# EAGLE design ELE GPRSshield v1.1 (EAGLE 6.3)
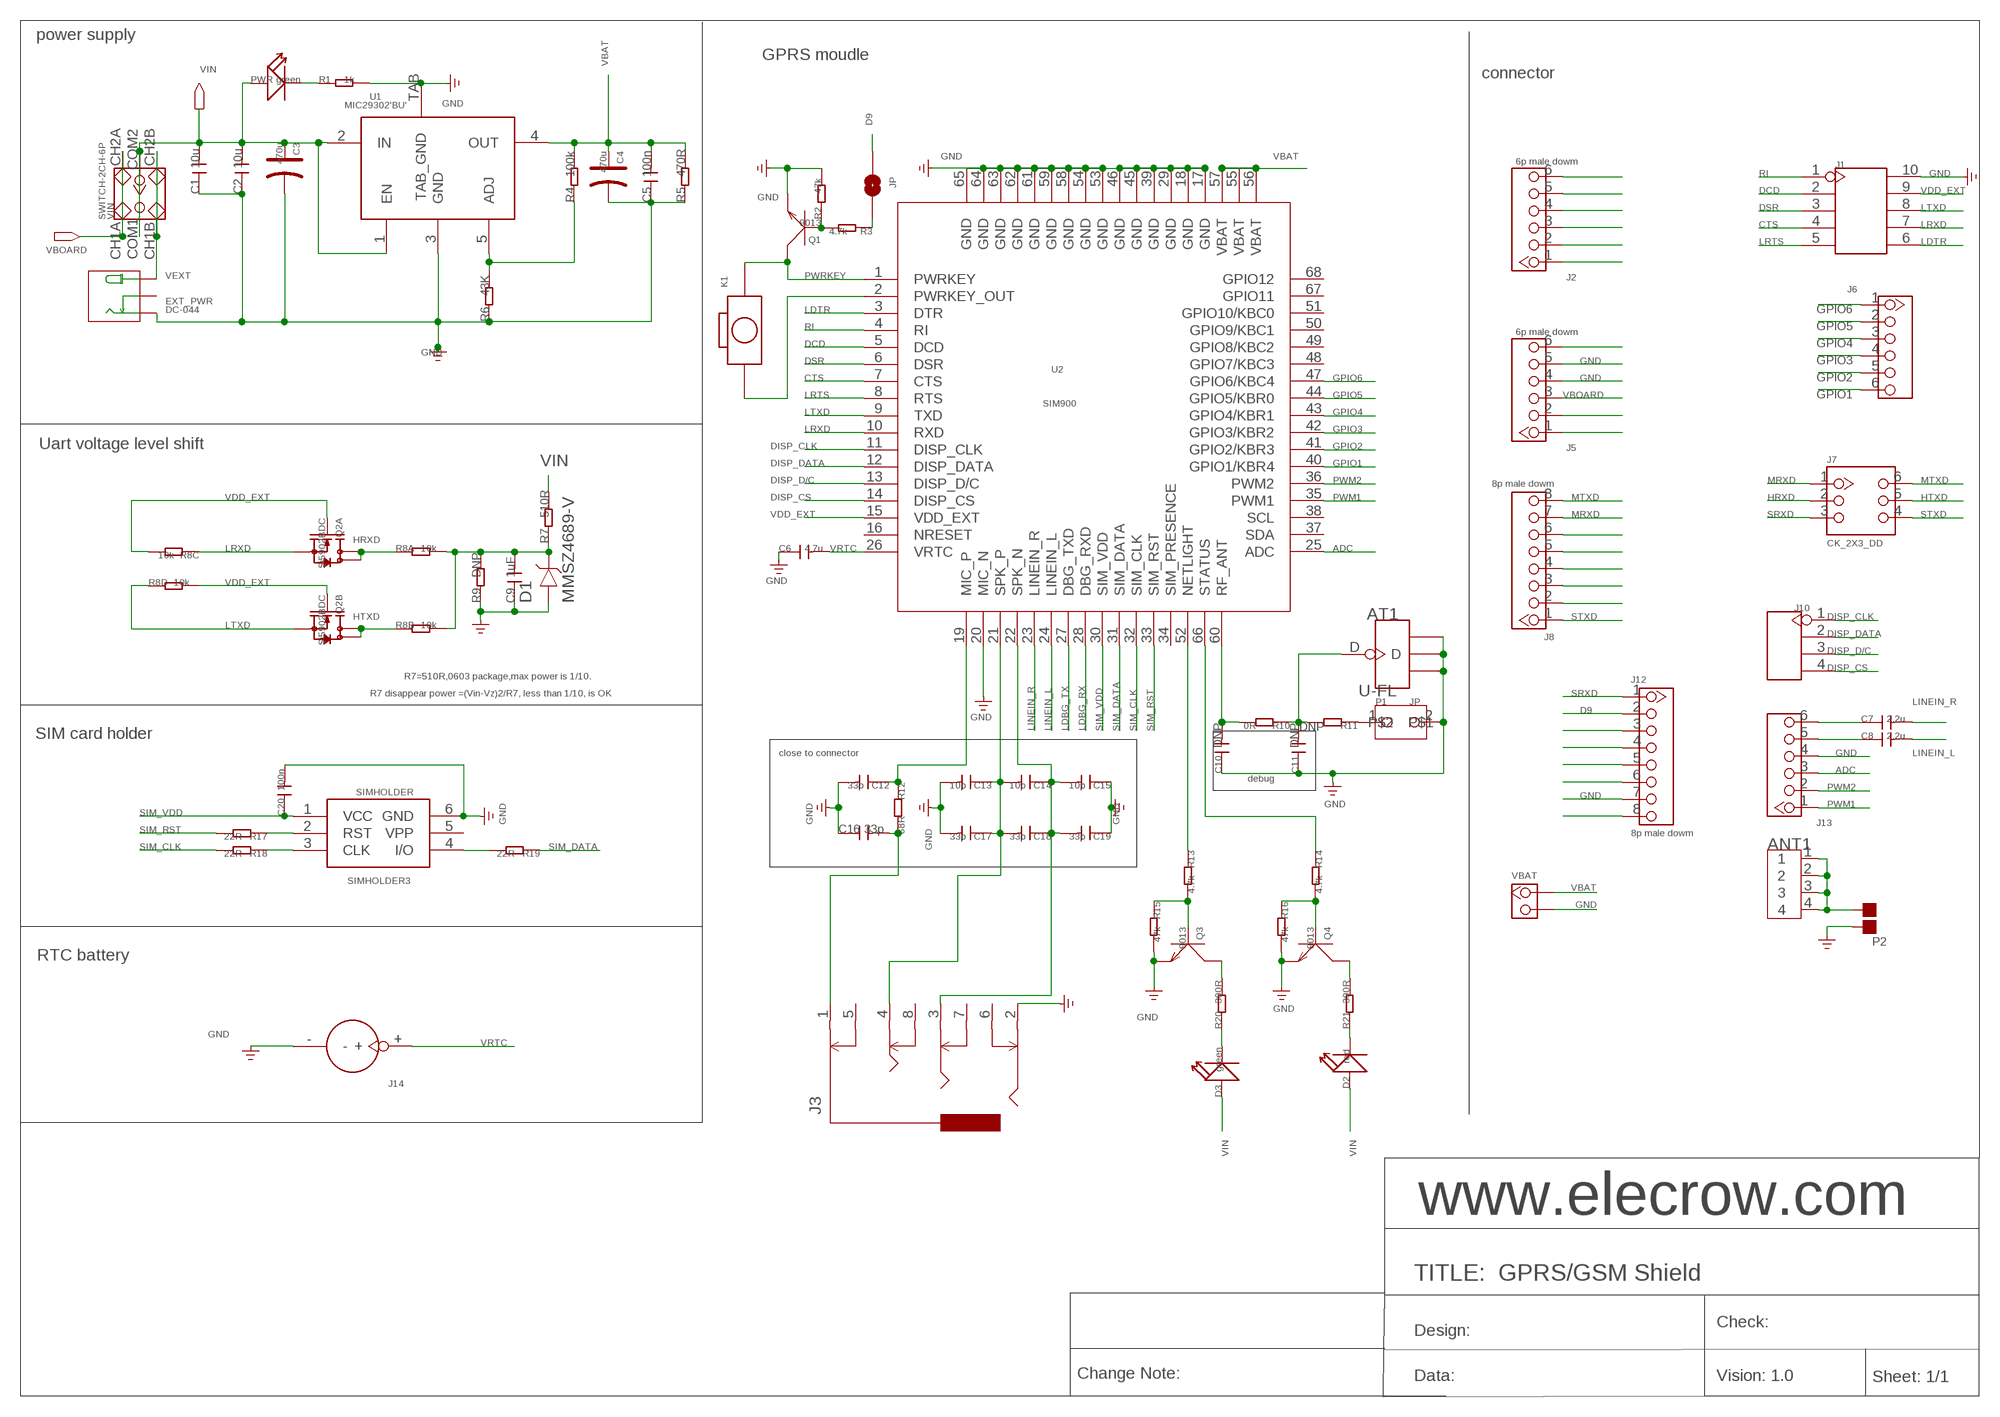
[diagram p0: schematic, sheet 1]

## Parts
ANT1  ANTENNA-SMA-IPX  [SMA-TO-IPX]
AT1  U-FL  ANTENNA-U-FL  [4P-U-FL]
C1  10u  C-0603  [0603]
C2  10u  C-0603  [0603]
C3  470u  006-CAP_AVX_D  [AVX_D]
C4  470u  006-CAP_AVX_D  [AVX_D]
C5  100n  C-0603  [0603]
C6  4.7u  C-0805  [0805]
C7  2.2u  C-0603  [0603]
C8  2.2u  C-0603  [0603]
C9  1uF  C-0603  [0603]
C10  DNP  C-0402  [0402]
C11  DNP  C-0402  [0402]
C12  33p  C-0603  [0603]
C13  10p  C-0402  [0402]
C14  10p  C-0402  [0402]
C15  10p  C-0402  [0402]
C16  33p  C-0603  [0603]
C17  33p  C-0402  [0402]
C18  33p  C-0402  [0402]
C19  33p  C-0402  [0402]
C20  100n  C-0603  [0603]
D1  MMSZ4689-V  D-VOL'MMSZ4681'  [SOD123-2.7X1.6]
D2  red  LED'0603'  [LED-0603]
D3  green  LED'0603'  [LED-0603]
EXT_PWR  DC-044  [DC-404]
J1  HEADER-2X5P-2.54  [2X5P-2.54]
J2  6p male dowm  HEADER_1X6  [CK_1X6]
J3  AUDIO-8P'PJ-3536-L6S'  [8P-3.5-SMD]
J5  6p male dowm  HEADER_1X6  [CK_1X6]
J6  HEADER_1X6  [CK_1X6]
J7  CK_2X3_DD  [CK_2X3]
J8  8p male dowm  CK_1X8DD  [CK_1X8]
J10  HEADER-4P'2.54-90D-FEMALE'  [4P-2.54-90D-FEMALE]
J12  8p male dowm  CK_1X8DD  [CK_1X8]
J13  HEADER_1X6  [CK_1X6]
J14  HOLDER-BATTERY-2P-CR1220  [CR1220]
JP  PAD-SOLDERJUMPERNC  [2P-SMD-3.3X2]
K1  BOTTON_1_DP  [BTN_5.0_RST]
P1  JP  [JP]
P2  PAD-JUMPER-2P  [2P-SMD-1.78X1.27]
PWR  green  007-LED0603  [D0603]
Q1  9013  TRANSISTOR-NPN-SOT23  [SOT23]
Q2  Si5902BDC  010-DUAL-N-MOSFET_1206-8  [1206-8]
Q3  9013  TRANSISTOR-NPN-SOT23  [SOT23]
Q4  9013  TRANSISTOR-NPN-SOT23  [SOT23]
R1  1k  R-0603  [0603]
R2  47k  R-0603  [0603]
R3  4.7k  R-0603  [0603]
R4  100k  R-0603  [0603]
R5  470R  R-0603  [0603]
R6  43K  R-0603  [0603]
R7  510R  R-0603  [0603]
R8  10k  R-4R-1206  [1206-8-3.3X2.4]
R9  DNP  R-0603  [0603]
R10  0R  R-0402  [0402]
R11  DNP  R-0402  [0402]
R12  68R  R-0603  [0603]
R13  4.7k  R-0603  [0603]
R14  4.7k  R-0603  [0603]
R15  47k  R-0603  [0603]
R16  47k  R-0603  [0603]
R17  22R  R-0603  [0603]
R18  22R  R-0603  [0603]
R19  22R  R-0603  [0603]
R20  300R  R-0603  [0603]
R21  300R  R-0603  [0603]
SIMHOLDER  SIMHOLDER3  [SIMHOLDER3]
U1  MIC29302'BU'  [TO-263]
U2  SIM900  ICS_V54_SIM900  [ICS_V54_SIM900]
VBAT  DNP  HEADER_1X2_2.54  [CK_1*2]
VIN  SWITCH-2CH-6P  [6P-2CH-2.54-7.6X3.0]

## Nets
ADC: J13.3 U2.25(ADC)
CTS: J1.4 U2.7(CTS)
D9: J12.2 JP.1
DCD: J1.2 U2.5(DCD)
DISP_CLK: J10.1 U2.11(DISP_CLK)
DISP_CS: J10.4 U2.14(DISP_CS)
DISP_D/C: J10.3 U2.13(DISP_D/C)
DISP_DATA: J10.2 U2.12(DISP_DATA)
DSR: J1.3 U2.6(DSR)
GND: AT1.GND1 AT1.GND2 AT1.GND3 C1.1 C2.1 C3.- C4.- C5.1 C6.1 C9.1 C10.1 C11.1 C12.2 C13.2 C15.1 C16.1 C17.2 C19.1 C20.2 D1.1 EXT_PWR.- J1.10 J3.2 J5.4 J5.5 J12.7 J13.4 J14.- P1.2 P2.2 Q1.2(E) Q3.2(E) Q4.2(E) R1.2 R2.2 R5.1 R6.1 R9.1 R15.2 R16.2 SIMHOLDER.6(GND) U1.3(GND) U1.TAB(TAB_GND) U2.17(GND) U2.18(GND) U2.20(MIC_N) U2.29(GND) U2.39(GND) U2.45(GND) U2.46(GND) U2.53(GND) U2.54(GND) U2.58(GND) U2.59(GND) U2.61(GND) U2.62(GND) U2.63(GND) U2.64(GND) U2.65(GND) VBAT.2
GPIO1: J6.6 U2.40(GPIO1/KBR4)
GPIO2: J6.5 U2.41(GPIO2/KBR3)
GPIO3: J6.4 U2.42(GPIO3/KBR2)
GPIO4: J6.3 U2.43(GPIO4/KBR1)
GPIO5: J6.2 U2.44(GPIO5/KBR0)
GPIO6: J6.1 U2.47(GPIO6/KBC4)
HRXD: J7.2 Q2.7(A:D) Q2.8(A:D) R8.1
HTXD: J7.5 Q2.5(B:D) Q2.6(B:D) R8.2
LDBG_RX: U2.28(DBG_RXD)
LDBG_TX: U2.27(DBG_TXD)
LDTR: J1.6 U2.3(DTR)
LINEIN_L: C8.2 U2.24(LINEIN_L)
LINEIN_R: C7.2 U2.23(LINEIN_R)
LRTS: J1.5 U2.8(RTS)
LRXD: J1.7 Q2.1(A:S) R8.3 U2.10(RXD)
LTXD: J1.8 Q2.3(B:S) R8.4 U2.9(TXD)
MRXD: J7.1 J8.7
MTXD: J7.6 J8.8
N$1: C10.2 R10.2 U2.60(RF_ANT)
N$2: R4.1 R6.2 U1.5(ADJ)
N$3: Q3.3(C) R20.2
N$4: R19.2 SIMHOLDER.4(I/O)
N$5: R18.1 SIMHOLDER.3(CLK)
N$6: R17.1 SIMHOLDER.2(RST)
N$7: D3.- R20.1
N$8: Q3.1(B) R13.2 R15.1
N$9: C9.2 D1.2 R7.1 R8.7 R8.8 R9.2
N$10: R13.1 U2.52(NETLIGHT)
N$11: K1.P$1 U2.2(PWRKEY_OUT)
N$12: ANT1.1 ANT1.2 ANT1.3 ANT1.4 P2.1
N$13: C12.1 R12.1 U2.19(MIC_P)
N$14: JP.2 R3.1
N$15: C13.1 C14.2 C17.1 C18.2 J3.4 U2.21(SPK_P)
N$16: Q4.3(C) R21.2
N$17: D2.- R21.1
N$18: Q4.1(B) R14.2 R16.1
N$19: C14.1 C15.2 C18.1 C19.2 J3.3 U2.22(SPK_N)
N$20: R14.1 U2.66(STATUS)
N$21: AT1.D C11.2 R10.1 R11.2
N$22: P1.1 R11.1
N$23: C7.1 J13.6
N$24: J8.6
N$25: J8.5
N$26: J8.4
N$27: J8.3
N$28: J8.2
N$29: C8.1 J13.5
N$30: C16.2 J3.1 R12.2
N$31: J2.6
N$32: J12.3
N$33: J12.4
N$34: J12.5
N$35: J12.6
N$36: Q1.1(B) R2.1 R3.2
N$37: J12.8
N$38: J2.5
N$41: J2.4
N$42: J2.3
N$43: J2.2
N$44: J2.1
N$45: J5.6
N$49: J5.2
N$50: J5.1
N$53: PWR.- R1.1
PWM1: J13.1 U2.35(PWM1)
PWM2: J13.2 U2.36(PWM2)
PWRKEY: K1.P$2 Q1.3(C) U2.1(PWRKEY)
RI: J1.1 U2.4(RI)
SIM_CLK: R18.2 U2.32(SIM_CLK)
SIM_DATA: R19.1 U2.31(SIM_DATA)
SIM_RST: R17.2 U2.33(SIM_RST)
SIM_VDD: C20.1 SIMHOLDER.1(VCC) U2.30(SIM_VDD)
SRXD: J7.3 J12.1
STXD: J7.4 J8.1
VBAT: C4.+ C5.2 R4.2 R5.2 U1.4(OUT) U2.55(VBAT) U2.56(VBAT) U2.57(VBAT) VBAT.1
VBOARD: J5.3 VIN.CH1A VIN.CH2A
VDD_EXT: J1.9 Q2.2(A:G) Q2.4(B:G) R8.5 R8.6 U2.15(VDD_EXT)
VEXT: EXT_PWR.+ VIN.CH1B VIN.CH2B
VIN: C1.2 C2.2 C3.+ D2.+ D3.+ PWR.+ R7.2 U1.1(EN) U1.2(IN) VIN.COM1 VIN.COM2
VRTC: C6.2 J14.+ U2.26(VRTC)
Unconnected: EXT_PWR.CDN J3.5 J3.6 J3.7 J3.8 SIMHOLDER.5(VPP) U2.16(NRESET) U2.34(SIM_PRESENCE) U2.37(SDA) U2.38(SCL) U2.48(GPIO7/KBC3) U2.49(GPIO8/KBC2) U2.50(GPIO9/KBC1) U2.51(GPIO10/KBC0) U2.67(GPIO11) U2.68(GPIO12)

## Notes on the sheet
- power supply
- GPRS moudle
- connector
- Uart voltage level shift
- R7=510R,0603 package,max power is 1/10.
- R7 disappear power =(Vin-Vz)2/R7, less than 1/10, is OK
- SIM card holder
- close to connector
- debug
- RTC battery
- www.elecrow.com
- TITLE:  GPRS/GSM Shield
- Check:
- Design:
- Change Note: | Data: | Vision: 1.0 | Sheet: 1/1

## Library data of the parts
ANT1 = Connector:ANTENNA-SMA-IPX
AT1 = Connector:ANTENNA-U-FL
C1 C2 C5-C20 = Discrete:C*: Ceramic Capacitors
C3 C4 = Discrete:006-CAP*: Electrolytic Capacitors,Tantalum Capacitors and Super Capacitors
D1 = template:D-VOL
D2 D3 = Discrete:LED*
EXT_PWR = Connector:DC-044
J1 = Connector:HEADER-2X5P
J2 J5 J6 J13 = CONNECTER:HEADER_1X6
J3 = template:AUDIO-8P
J7 = CONNECTER:CK_2X3
J8 J12 = CONNECTER:CK_1X8
J10 = Connector:HEADER-4P
J14 = Connector:HOLDER-BATTERY-2P
JP = Discrete:PAD-SOLDERJUMPER: Solder Jumper
K1 = CPT_SMD:BOTTON_1
P1 = mySeeed:JP
P2 = Discrete:PAD-JUMPER-2P; PARTNO: DNP
PWR = Discrete:007-LED*
Q1 Q3 Q4 = Discrete:TRANSISTOR-NPN*: NPN audion
Q2 = Discrete:010-DUAL-N-MOSFET*: Si5902BDC Si5904DC Si5908DC Si5920DC
R1-R7 R9-R21 = Discrete:R*
R8 = Discrete:R-4R*: Resistor Array
SIMHOLDER = SparkFun2:SIMHOLDER3
U1 = ICs_v54:MIC29302
U2 = Elecrow_test:ICS_V54_SIM900
VBAT = CONNECTER:HEADER_1X2
VIN = Discrete:SWITCH-2CH-6P

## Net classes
0 default: clearance 0.152 mm

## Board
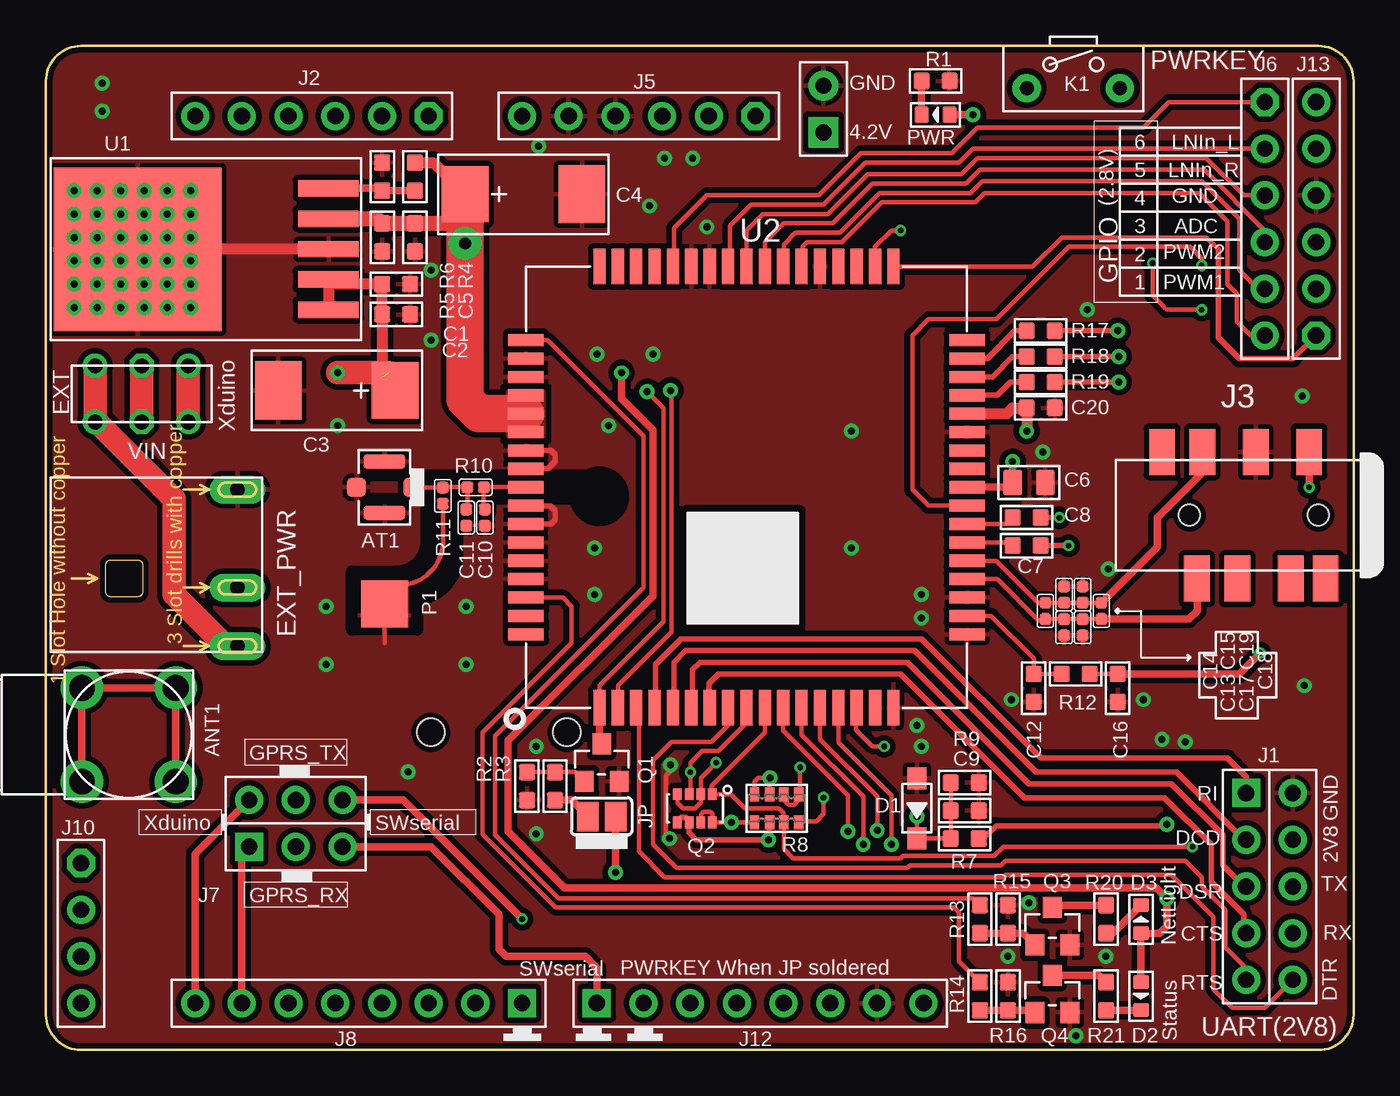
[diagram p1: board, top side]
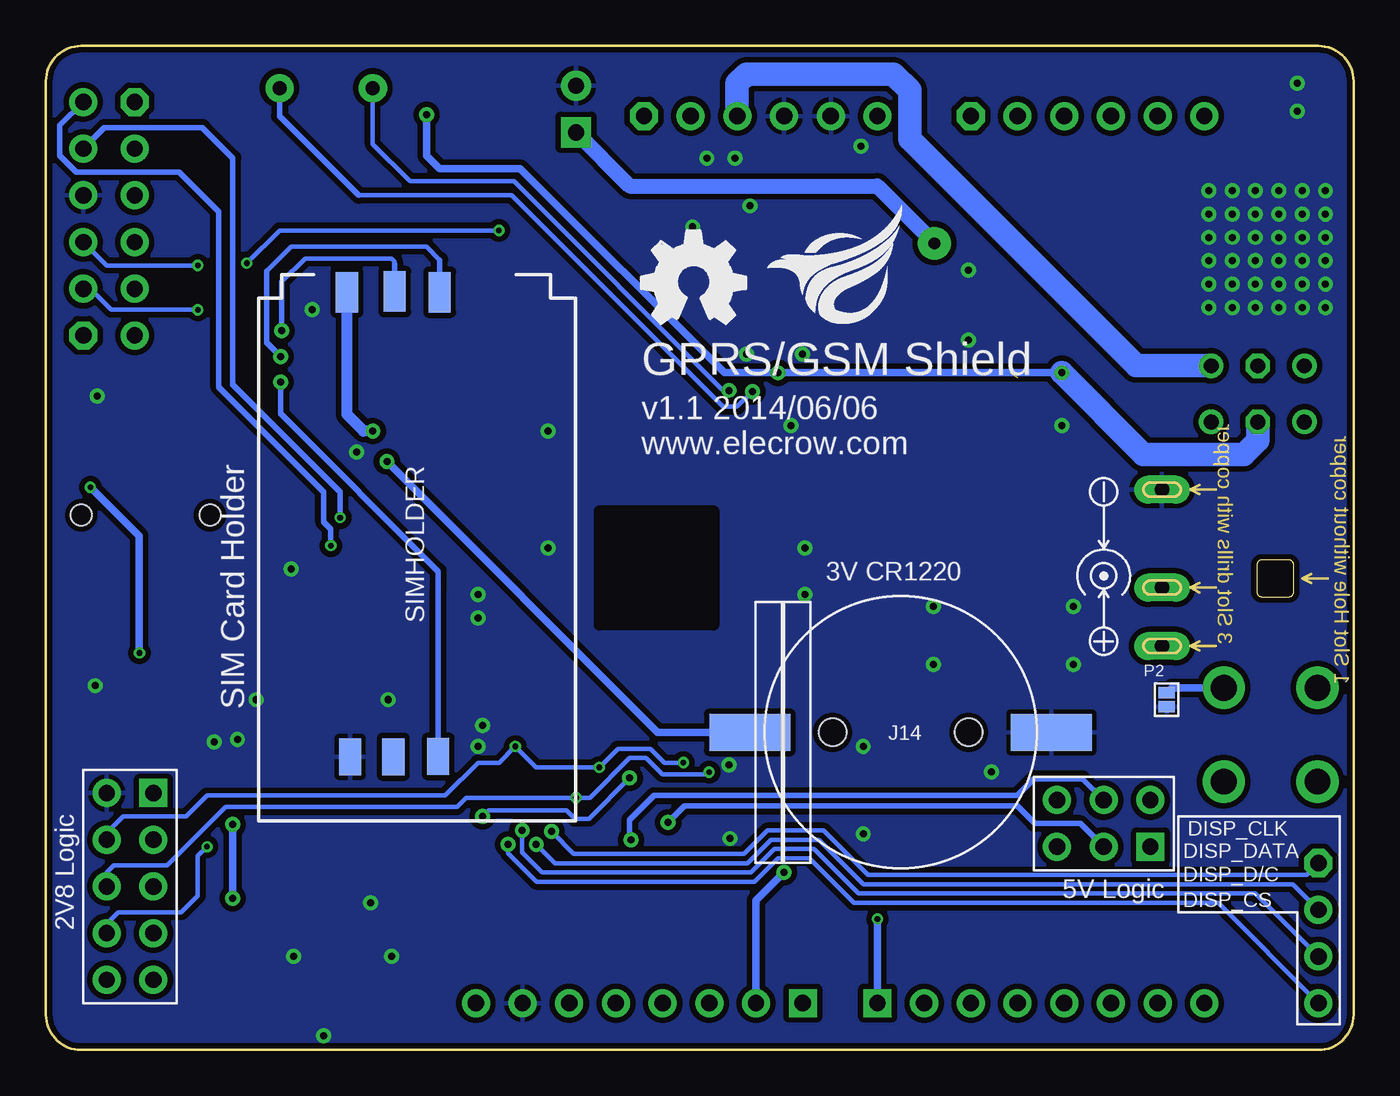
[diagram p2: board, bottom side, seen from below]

Size 71.12 x 54.61 mm. Coordinates in mm from the lower left corner, seen from the top.
Outline: 1.91,54.61 69.22,54.61 arc-90 71.12,52.7 71.12,1.91 arc-90 69.22,0 1.91,0 arc-90 0,1.91 0,52.7 arc-90 1.91,54.61
Copper layers (1*16): Top 0.035mm / dielectric 1.5mm / Bottom 0.035mm
Design rules "default *": minimum track width 6mil, minimum drill 12mil, track to track 6mil, track to pad 6mil, pad to pad 6mil, via to via 6mil, smd to smd 0mil, copper to edge 10mil, drill to drill 10mil, minimum pad ring 10mil, minimum via ring 6mil, stop-mask expansion 2mil, vias tented up to drill 100mil, thermal gap 10mil
tRestrict: area 34.8,23.1 to 41,29.3; area 35.6,41.9 to 35.7,43.3; area 25.5,37 to 26.7,37.2; area 25.7,32 to 26.5,32.1; area 25.7,28.1 to 26.5,28.2; area 25.7,27.1 to 26.5,27.2; area 25.7,26 to 26.5,26.2; area 25.7,29.1 to 26.4,29.2; 11 lines
bRestrict: area 34.8,23.1 to 41,29.3

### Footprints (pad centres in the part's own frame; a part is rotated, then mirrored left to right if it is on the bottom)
SMA-TO-IPX = drill 1.4 pad 2.3: 1 -2.55,2.55; 2 2.55,2.55; 3 2.55,-2.55; 4 -2.55,-2.55
U-FL = smd 1.016 x 1.016: D -1.524,0; GND3 1.524,0 | smd 2.286 x 0.762: GND1 0,1.397; GND2 0,-1.397
0603 = smd 0.889 x 0.889: 1 -0.762,0; 2 0.762,0
AVX_D = smd 2.54 x 3.048: + -3.175,0 | smd 2.54 x 3.175: - 3.175,0
0805 = smd 1.016 x 1.397: 1 -0.889,0; 2 0.889,0
0603@1 = smd 0.889 x 0.889: 1 -0.762,0; 2 0.762,0
0402@1 = smd 0.635 x 0.635: 1 -0.445,0; 2 0.445,0
SOD123-2.7X1.6 = smd 1.2 x 1.02: 1 -1.635,0; 2 1.635,0
D0603 = smd 0.762 x 0.889: + -0.762,0; - 0.762,0
DC-404 = drill 0.813 pad 1.524 long: + 3.175,10.16; - -5.334,10.16; CDN 0,10.16
2X5P-2.54-LEADED = drill 0.889 pad 1.524 square: 1 -1.27,5.08 | drill 0.889 pad 1.524: 2 -1.27,2.54; 3 -1.27,0; 4 -1.27,-2.54; 5 -1.27,-5.08; 6 1.27,-5.08; 7 1.27,-2.54; 8 1.27,0; 9 1.27,2.54; 10 1.27,5.08
CK_1X6 = drill 0.889 pad 1.524 octagon: 1 0,6.35 | drill 0.889 pad 1.524: 2 0,3.81; 3 0,1.27; 4 0,-1.27; 5 0,-3.81; 6 0,-6.35
8P-3.5-SMD = smd 1.4 x 2.5: 1 2.8,-3.45; 2 5.7,-3.45; 3 8.6,-3.45; 4 8.9,3.45; 5 1.9,3.45; 6 3.8,3.45; 7 6.7,3.45; 8 10.8,-3.45 | hole 1.149: 2.3,0; 9.3,0
CK_2X3 = drill 0.889 pad 1.524 square: 1 -1.27,2.54 | drill 0.889 pad 1.524: 2 -1.27,0; 3 -1.27,-2.54; 4 1.27,-2.54; 5 1.27,0; 6 1.27,2.54
CK_1X8 = drill 0.889 pad 1.524 square: 1 0,8.89 | drill 0.889 pad 1.524: 2 0,6.35; 3 0,3.81; 4 0,1.27; 5 0,-1.27; 6 0,-3.81; 7 0,-6.35; 8 0,-8.89
4P-2.54 = drill 0.889 pad 1.524 octagon: 1 0,3.81 | drill 0.889 pad 1.524: 2 0,1.27; 3 0,-1.27; 4 0,-3.81
CR1220 = smd 2 x 4.4: + 0,-8.2; - 0,8.2 | hole 1.5: 0,3.7; 0,-3.7
2P-SMD-3.3X2 = smd 1.168 x 1.6: 1 -0.762,0; 2 0.762,0
BTN_5.0_RST = drill 0.762 pad 1.524: P$1 0,2.54; P$2 0,-2.54
JP = smd 1.27 x 2.54: 1 -0.635,0; 2 0.635,0
2P-SMD-1.78X1.27 = smd 0.889 x 0.61: 1 0,0.381; 2 0,-0.381
SOT23 = smd 1.016 x 1.143: 1 -0.95,-1.016; 2 0.95,-1.016; 3 0,1.016
1206-8 = smd 0.457 x 0.635: 1 -0.953,-0.762; 2 -0.318,-0.762; 3 0.318,-0.762; 4 0.953,-0.762; 5 0.953,0.762; 6 0.318,0.762; 7 -0.318,0.762; 8 -0.953,0.762
1206-8-3.3X2.4 = smd 0.508 x 0.762: 1 -1.206,-0.762; 2 -0.381,-0.762; 3 0.381,-0.762; 4 1.206,-0.762; 5 1.206,0.762; 6 0.381,0.762; 7 -0.381,0.762; 8 -1.206,0.762
0402 = smd 0.635 x 0.635: 1 -0.445,0; 2 0.445,0
SIMHOLDER3 = smd 2.2 x 1.2: 1 0.95,4.81; 2 0.91,7.41; 3 0.95,9.86 | smd 2 x 1.2: 4 26.2,9.78; 5 26.22,7.34; 6 26.22,4.98
TO-263 = smd 3.302 x 0.889: 1 3.302,-3.302; 2 3.302,-1.651; 3 3.302,0; 4 3.302,1.651; 5 3.302,3.302 | smd 9.12 x 8.89: TAB -7.071,-0.03
ICS_V54_SIM900 = smd 1.93 x 0.66: 1 -12,8; 2 -12,7; 3 -12,6; 4 -12,5; 5 -12,4; 6 -12,3; 7 -12,2; 8 -12,1; 9 -12,0; 10 -12,-1; 11 -12,-2; 12 -12,-3; 13 -12,-4; 14 -12,-5; 15 -12,-6; 16 -12,-7; 17 -12,-8; 35 12,-8; 36 12,-7; 37 12,-6; 38 12,-5; 39 12,-4; 40 12,-3; 41 12,-2; 42 12,-1; 43 12,0; 44 12,1; 45 12,2; 46 12,3; 47 12,4; 48 12,5; 49 12,6; 50 12,7; 51 12,8 | smd 0.66 x 1.93: 18 -8,-12; 19 -7,-12; 20 -6,-12; 21 -5,-12; 22 -4,-12; 23 -3,-12; 24 -2,-12; 25 -1,-12; 26 0,-12; 27 1,-12; 28 2,-12; 29 3,-12; 30 4,-12; 31 5,-12; 32 6,-12; 33 7,-12; 34 8,-12; 52 8,12; 53 7,12; 54 6,12; 55 5,12; 56 4,12; 57 3,12; 58 2,12; 59 1,12; 60 0,12; 61 -1,12; 62 -2,12; 63 -3,12; 64 -4,12; 65 -5,12; 66 -6,12; 67 -7,12; 68 -8,12
CK_1*2 = drill 0.889 pad 1.651 square: 1 0,1.27 | drill 0.889 pad 1.651: 2 0,-1.27
6P-2CH-2.54-7.6X3.0 = drill 0.813 pad 1.27: CH1A -1.524,2.54; CH1B -1.524,-2.54; CH2A 1.524,2.54; CH2B 1.524,-2.54 | drill 0.813 pad 1.27 octagon: COM1 -1.524,0; COM2 1.524,0

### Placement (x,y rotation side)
ANT1  4.51,17.14 270 top
AT1  U-FL  [U-FL]  18.41,30.61 180 top
C1  19.05,41.66 180 top
C2  19.05,40.01 180 top
C3  15.81,35.88 180 top
C4  25.97,46.55 0 top
C5  20.07,44.2 90 top
C6  53.47,30.86 180 top
C7  2.2u  [0603@1]  53.34,27.43 180 top
C8  2.2u  [0603@1]  53.34,28.96 180 top
C9  49.97,13.02 180 top
C10  DNP  [0402@1]  23.88,28.96 90 top
C11  DNP  [0402@1]  22.86,28.96 90 top
C12  53.72,19.68 270 top
C13  10p  [0402@1]  55.37,22.99 270 top
C14  10p  [0402@1]  54.36,23.88 270 top
C15  10p  [0402@1]  55.37,24.77 270 top
C16  58.29,19.68 90 top
C17  33p  [0402@1]  56.39,22.99 270 top
C18  33p  [0402@1]  57.4,23.88 270 top
C19  33p  [0402@1]  56.39,24.77 270 top
C20  54.1,34.92 0 top
D1  47.37,13.14 270 top
D2  red  [D0603]  59.56,2.92 270 top
D3  green  [D0603]  59.56,7.11 90 top
EXT_PWR  0.25,25.15 270 top
J1  [2X5P-2.54-LEADED]  66.55,8.89 0 top
J2  14.46,50.8 270 top
J3  71.5,29.08 180 top
J5  32.24,50.8 270 top
J6  66.29,45.21 0 top
J7  13.59,12.32 90 top
J8  17,2.54 270 top
J10  [4P-2.54]  1.91,6.35 0 top
J12  38.85,2.54 90 top
J13  69.09,45.21 180 top
J14  24.64,17.27 270 bottom
JP  30.23,12.7 180 top
K1  55.88,52.32 90 top
LOGO2  LOGO-OSHW-FILLX0200-NT  [OSHW_FILLX200_NOTEXT]  38.73,39.5 0 bottom
P1  18.41,24.26 270 top
P2  10.16,19.05 0 bottom
PWR  48.39,50.86 180 top
Q1  30.23,15.62 0 top
Q2  35.3,13.14 180 top
Q3  54.74,6.73 0 top
Q4  54.74,3.05 0 top
R1  1k  [0603@1]  48.39,52.7 0 top
R2  26.16,14.35 270 top
R3  27.69,14.35 90 top
R4  20.07,47.5 90 top
R5  18.29,44.2 90 top
R6  18.29,47.5 270 top
R7  49.97,11.49 0 top
R8  39.74,13.14 0 top
R9  49.97,14.54 180 top
R10  23.37,30.61 0 top
R11  21.59,30.15 90 top
R12  56.01,20.45 0 top
R13  50.8,7.11 270 top
R14  50.8,2.92 270 top
R15  52.32,7.11 90 top
R16  52.32,2.92 90 top
R17  54.1,39.12 180 top
R18  54.1,37.72 180 top
R19  54.1,36.32 0 top
R20  57.66,7.11 90 top
R21  57.66,2.92 90 top
SIMHOLDER  59.56,42.16 270 bottom
U1  12.06,43.56 0 top
U2  38.1,30.61 90 top
U$4  [ELECROW_NRW_6]  31.88,39.5 0 bottom
VBAT  42.29,51.18 180 top
VIN  5.21,35.69 270 top

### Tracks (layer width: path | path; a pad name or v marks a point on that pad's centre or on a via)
ADC  (via drill 0.3 pad 0.41)
  Top 0.254: U2.25 47.99,29.61 47.12,30.48 47.12,38.86 48.01,39.75 51.69,39.75 55.5,43.56 55.63,43.69 62.23,43.69 62.87,43.05 v62.87,42.67
  Bottom 0.254: v62.87,42.67 67.82,42.67 J13.3
CTS
  Top 0.305: 65.15,6.35 J1.4 65.15,6.48 65.15,7.37 63.37,9.14 63.37,11.18 60.83,13.72 53.21,13.72 46.48,20.45 36.58,20.45 36.07,19.94 36.07,18.64 U2.7
D9  (via drill 0.38 pad 0.81)
  Top 0.406: v30.99,9.65 JP.1
  Bottom 0.406: v30.99,9.65 32.5,8.14 J12.2
DCD
  Top 0.305: J1.2 65.15,11.43 61.47,15.11 53.85,15.11 47.24,21.72 34.8,21.72 34.16,21.08 34.16,18.67 U2.5
DISP_CLK  (via drill 0.38 pad 0.81)
  Top 0.254: U2.11 40.1,17.37 43.62,13.84 v43.62,11.87
  Bottom 0.254: J10.1 2.54,9.53 26.42,9.53 28.83,11.94 31.88,11.94 33.15,10.67 42.42,10.67 v43.62,11.87
DISP_CS  (via drill 0.38 pad 0.81)
  Top 0.254: U2.14 43.1,16.72 45.97,13.84 v45.97,11.18
  Bottom 0.254: v45.97,11.18 45.97,10.68 44.44,9.14 32.58,9.14 31.3,10.41 29.59,10.41 27.18,8 7.37,8 J10.4
DISP_D/C  (via drill 0.38 pad 0.81)
  Top 0.254: U2.13 42.1,16.89 45.21,13.78 v45.21,11.94
  Bottom 0.254: v45.21,11.94 45.21,10.74 44.13,9.65 32.77,9.65 31.5,10.92 29.34,10.92 26.92,8.51 5.33,8.51 J10.3
DISP_DATA  (via drill 0.38 pad 0.81)
  Top 0.254: U2.12 41.1,17.13 44.45,13.78 v44.45,11.18
  Bottom 0.254: J10.2 3.3,9.02 26.67,9.02 29.08,11.43 31.69,11.43 32.96,10.16 43.43,10.16 v44.45,11.18
DSR
  Top 0.305: J1.3 65.15,8.89 64.01,10.03 64.01,11.68 61.21,14.48 53.47,14.48 46.86,21.08 35.56,21.08 35.18,20.7 35.18,18.69 U2.6
GND  (via drill 0.38 pad 0.81)
  Top 0.254: 18.41,22.15 P1.2 | v33.97,15.49 33.97,15.18 33.72,14.92 33.72,11.68 v33.91,11.49
  Top 0.305: U2.62 27.46,28.61 27.69,28.83 27.69,29.34 27.43,29.59 26.12,29.59 U2.61 | U2.58 27.46,32.61 27.69,32.38 27.69,32 27.3,31.62 26.12,31.62 U2.59
  Top 0.61: U1.3 8.51,43.56 v7.87,42.93
  Top 0.813: 8.74,43.43 arc-45 8.56,43.51 v7.87,44.2
  other vias: 47.62,24.77 57.78,26.16 60.71,16.89 68.45,19.81 47.62,16.51 68.33,35.56 56.64,40.26 7.87,40.39 7.87,41.66 7.87,45.47 7.87,46.74 6.6,46.74 5.33,46.74 4.06,46.74 2.79,46.74 1.52,46.74 1.52,45.47 1.52,44.2 1.52,42.93 1.52,41.66 1.52,40.39 4.06,45.47 4.06,44.2 4.06,42.93 4.06,41.66 4.06,40.39 2.79,45.47 2.79,44.2 2.79,42.93 2.79,41.66 2.79,40.39 5.33,45.47 5.33,44.2 5.33,42.93 5.33,41.66 5.33,40.39 6.6,45.47 6.6,44.2 6.6,42.93 6.6,41.66 6.6,40.39 54.23,32.51 61.98,16.76 22.86,20.95 26.67,11.75 53.47,8 57.66,5.08 52.32,5.08 56.01,0.76 19.68,15.11 20.95,42.42 20.95,38.61 26.8,49.15 32.83,45.91 3.05,51.05 3.05,52.58 29.97,37.85 33.02,37.85 35.94,44.77 43.81,33.66 43.81,27.3 33.66,48.51 35.18,48.51 47.37,17.65 26.67,16.51 30.61,33.97 29.84,24.77 29.84,27.3 22.86,24.13 15.88,33.97 15.24,24.13 15.24,20.95 47.62,23.5 52.51,19.05 59.69,19.05
  pour Bottom (isolate 0.305): -0.51,54.99 71.5,55.24 71.5,-0.25 -1.14,-0.38
  pour Top (isolate 0.305, rank 6): -0.51,55.12 71.75,55.24 71.5,-0.51 -1.02,-0.38
GPIO1
  Top 0.254: J6.6 65.53,38.86 64.77,39.62 64.77,41.15 64.26,41.66 64.26,45.09 62.74,46.61 51.05,46.61 50.55,46.1 45.47,46.1 43.31,43.94 41.4,43.94 41.15,43.69 41.15,42.66 U2.40
GPIO2
  Top 0.254: J6.5 65.91,41.4 64.9,42.42 64.9,45.21 62.87,47.24 50.93,47.24 50.29,46.61 45.34,46.61 43.18,44.45 40.77,44.45 40.13,43.81 40.13,42.64 U2.41
GPIO3
  Top 0.254: J6.4 66.29,44.58 62.99,47.88 50.8,47.88 50.04,47.12 44.96,47.12 42.8,44.96 40.13,44.96 39.12,43.94 39.12,42.62 U2.42
GPIO4
  Top 0.254: U2.43 38.1,44.58 38.99,45.47 42.55,45.47 44.7,47.62 49.78,47.62 50.67,48.51 63.12,48.51 65.15,46.48 J6.3
GPIO5
  Top 0.254: J6.2 50.42,49.02 49.66,48.26 44.58,48.26 42.29,45.97 38.35,45.97 37.21,44.83 37.21,42.72 U2.44
GPIO6
  Top 0.254: J6.1 61.09,51.56 59.69,50.16 50.67,50.16 49.28,48.77 44.32,48.77 42.04,46.48 35.94,46.48 34.16,44.7 34.16,42.67 U2.47
HRXD  (via drill 0.38 pad 0.81)
  Top 0.254: Q2.8 v37.27,12.38 R8.1 | Q2.8 36.25,12.44 | Q2.7 35.62,12.8 35.77,12.95 36.13,12.95 36.26,12.83 Q2.8
  Bottom 0.305: J7.2 14.86,12.32 17.34,12.32 18.29,13.27 36.39,13.27 v37.27,12.38
HTXD  (via drill 0.38 pad 0.81)
  Top 0.254: R8.2 39.36,11.48 v39.31,11.43
  Top 0.305: v39.31,11.43 35.37,11.43 34.98,11.82 Q2.6 34.98,12.45 34.8,12.64 34.54,12.64 34.34,12.44 Q2.5
  Bottom 0.305: J7.5 14.75,14.75 17.38,14.75 18.29,13.84 38.04,13.84 39.37,12.51 39.37,11.49 v39.31,11.43
LDTR
  Top 0.254: J1.6 66.29,2.29 64.52,2.29 63.5,3.3 63.5,7.24 61.21,9.53 52.2,9.53 52.07,9.4 33.66,9.4 32.26,10.79 32.26,18.45 U2.3
LINEIN_L
  Top 0.254: U2.24 52.23,28.61 C8.2
LINEIN_R
  Top 0.254: U2.23 52.4,27.61 C7.2
LRTS
  Top 0.254: J1.5 65.28,4.45 64.14,5.59 64.14,7.62 62.87,8.89 62.87,9.4 61.98,10.29 52.2,10.29 51.94,10.03 46.99,10.03 46.86,9.91 34.29,9.91 33.02,11.18 33.02,15.75 34.04,16.76 36.2,16.76 37.08,17.65 37.08,18.59 U2.8
LRXD  (via drill 0.3 pad 0.41)
  Top 0.254: U2.10 39.1,17.26 36.2,14.35 36.2,13.96 Q2.1 37.26,13.9 38.02,13.14 39.88,13.14 40.12,12.9 R8.3 40.13,12.37 40.13,10.92 40.64,10.41 46.48,10.41 46.61,10.54 51.56,10.54 52.07,11.05 v62.36,11.05
  Bottom 0.254: J1.7 67.82,6.86 67.18,7.49 65.79,7.49 65.28,7.49 63.75,7.49 62.87,8.38 62.87,10.54 v62.36,11.05
LTXD  (via drill 0.3 pad 0.41)
  Top 0.254: 40.95,12.44 R8.4 41.02,12.31 | 40.95,12.44 40.96,12.45 | Q2.3 35.05,13.98 v35.05,15.11 35.05,15.62 35.69,16.26 36.58,16.26 38.1,17.78 U2.9 | 40.95,12.44 41.9,12.44 42.29,12.83 v42.29,13.72
  Bottom 0.254: v35.05,15.11 35.18,14.99 37.59,14.99 38.48,15.88 39.37,15.88 41.53,13.72 v42.29,13.72 48.26,13.72 48.77,13.21 61.34,13.21 64.52,10.03 67.44,10.03 67.82,9.65 J1.8
MRXD
  Top 0.406: J7.1 10.65,10.65 J8.7
MTXD
  Top 0.406: J7.6 8.11,10.65 J8.8
N$1
  Top 0.254: U2.60 R10.2 23.81,29.46 C10.2
N$2
  Top 0.406: R4.1 R6.2 18.16,46.86 U1.5
N$3
  Top 0.406: R20.2 54.86,7.87 Q3.3
N$4  (via drill 0.38 pad 0.81)
  Top 0.305: v58.36,36.32 R19.2
  Bottom 0.254: 49.78,25.02
  Bottom 0.305: SIMHOLDER.4 49.78,25.02 | v58.36,36.32 58.36,34.61 49.78,26.04 49.78,25.02
N$5  (via drill 0.38 pad 0.81)
  Top 0.305: v58.36,37.72 R18.1
  Bottom 0.254: 59.12,42.35 57.78,43.69 50.42,43.69 49.7,42.97
  Bottom 0.305: SIMHOLDER.3 49.7,42.97 | 59.12,42.35 59.12,38.48 v58.36,37.72
N$6  (via drill 0.38 pad 0.81)
  Top 0.305: v58.29,39.12 R17.1
  Bottom 0.254: 52.15,42.76 52.15,42.88 52.32,43.05 57.02,43.05 58.29,41.78
  Bottom 0.305: SIMHOLDER.2 52.15,42.76 | v58.29,39.12 58.29,41.78
N$7
  Top 0.406: R20.1 58.04,6.35 D3.-
N$8
  Top 0.406: R13.2 R15.1 53.15,6.35 Q3.1
N$9  (via drill 0.38 pad 0.81)
  Top 0.254: R8.7 39.36,14.79 v39.37,14.8 38.73,14.8 38.54,14.6 R8.8 | v47.37,12.7 D1.2 49.2,11.51 R7.1 C9.2 R9.2
  Bottom 0.254: v39.37,14.8 41.59,12.57 42.35,12.57 42.8,13.02 47.05,13.02 v47.37,12.7
N$10
  Top 0.254: U2.52 27.29,38.61 32.51,33.39 32.51,25.15 24.44,17.07 24.44,11.7 27.89,8.26 50.42,8.26 R13.1
N$11  (via drill 0.38 pad 0.81)
  Top 0.254: U2.2 31.11,18.62 31.11,19.81 34.04,22.73 34.04,35.81 v33.97,35.88
  Bottom 0.254: v33.97,35.88 34.29,35.88 45.66,47.24 51.31,47.24 53.34,49.28 K1.P$1
N$12
  Top 0.406: ANT1.3 ANT1.4 ANT1.1 ANT1.2
  Bottom 0.406: ANT1.1 9.9,19.7 P2.1
N$13
  Top 0.254: U2.19 51.4,23.61 53.72,21.28 C12.1 R12.1
N$14
  Top 0.406: R3.1 28.57,13.59 JP.2
N$15
  Top 0.254: C18.2 C17.1 C13.1 C14.2 54.29,23.37 53.98,23.37 51.74,25.61 U2.21
  Top 0.406: C18.2 62.17,23.43 62.61,23.88 J3.4
N$16
  Top 0.406: Q4.3 57.28,4.06 R21.2
N$17
  Top 0.406: R21.1 D2.-
N$18
  Top 0.406: R14.2 R16.1 53.66,2.16 Q4.1
N$19
  Top 0.254: C18.1 C19.2 C15.2 C14.1 53.98,24.32 51.69,26.61 U2.22
  Top 0.406: C18.1 60.45,27.37 60.45,28.96 62.9,31.41 J3.3
N$20
  Top 0.254: U2.66 28.12,24.61 28.6,24.13 28.6,22.12 23.76,17.28 23.76,11.71 27.73,7.75 49.4,7.75 49.66,7.49 49.66,4.83 R14.1
N$21
  Top 0.254: AT1.D arc91 19.95,30.59 R11.2 arc-91 21.6,30.61 R10.1 22.92,29.46 C11.2
N$22
  Top 0.254: R11.1 21.59,27.56 arc-90 19.05,25.27 18.8,25.27 arc90 P1.1
N$23  (via drill 0.3 pad 0.41)
  Top 0.305: C7.1 v55.63,27.43
  Bottom 0.305: v55.63,27.43 55.63,28.32 56.01,28.7 56.01,30.35 61.72,36.07 61.72,45.59 63.88,47.75 69.47,47.75 70.36,48.64 70.36,50.29 J13.6
N$29  (via drill 0.3 pad 0.41)
  Top 0.305: C8.1 v55.12,28.96
  Bottom 0.305: v55.12,28.96 55.12,30.35 60.96,36.2 60.96,48.51 62.61,50.16 67.94,50.16 J13.5
N$30  (via drill 0.3 pad 0.41)
  Top 0.254: C16.2 R12.2
  Top 0.406: C16.2 64.9,20.45 v66.04,21.59 | v68.71,30.61 J3.1
  Bottom 0.406: v66.04,21.59 66.04,27.94 v68.71,30.61
N$36
  Top 0.254: R2.1 R3.2 28.77,15.11 Q1.1
N$53
  Top 0.406: PWR.- R1.1
PWM1
  Top 0.254: U2.35 53.66,42.61 55.24,44.2 63.12,44.2 63.75,43.56
  Top 0.305: 63.75,43.56 63.75,38.73 64.9,37.59 67.82,37.59 J13.1
PWM2  (via drill 0.3 pad 0.41)
  Top 0.254: 45.09,41.91 45.09,42.59 U2.36 45.1,43.7 45.97,44.58 v46.48,44.58 | v60.2,42.8 60.2,41.02 60.77,40.45 60.83,40.39 60.96,40.26 v62.87,40.26
  Bottom 0.254: J13.2 68.71,41.4 67.56,40.26 v62.87,40.26 | v46.48,44.58 58.42,44.58 v60.2,42.8
PWRKEY  (via drill 0.38 pad 0.81)
  Top 0.254: U2.1 30.1,19.81 33.59,23.3 33.59,34.92 v32.7,35.81
  Top 0.406: U2.1 30.1,16.76 Q1.3
  Bottom 0.254: v32.7,35.81 33.53,34.99 34.29,34.99 45.78,46.48 54.1,46.48
  Bottom 0.305: K1.P$2 58.42,50.8 54.1,46.48
RI
  Top 0.305: J1.1 65.28,14.86 64.26,15.88 54.1,15.88 47.62,22.35 34.54,22.35 33.15,20.95 33.15,18.65 U2.4
SIM_CLK
  Top 0.305: U2.32 51.47,36.61 52.58,37.72 R18.2
SIM_DATA
  Top 0.305: U2.31 51.74,35.61 52.45,36.32 R19.1
SIM_RST
  Top 0.305: U2.33 51.2,37.61 52.7,39.12 R17.2
SIM_VDD  (via drill 0.38 pad 0.81)
  Top 0.61: U2.30 52.26,34.61 52.58,34.92 C20.1 v53.34,33.66
  Bottom 0.61: SIMHOLDER.1 54.75,34.56 53.85,33.66 v53.34,33.66
SRXD
  Top 0.406: J7.3 20.95,11.05 24.64,7.37 24.64,5.46 25.02,5.08 29.34,5.08 29.97,4.45 29.97,2.55 J12.1
STXD  (via drill 0.3 pad 0.41)
  Top 0.406: v25.89,7.13 19.43,13.59 J7.4
  Bottom 0.406: v25.89,7.13 J8.1
VBAT  (via drill 0.64 pad 1.78)
  Top 0.406: 18.03,45.21 R5.2
  Top 0.61: R4.2 21.08,48.26 C4.+
  Top 0.813: U1.4 18.03,45.21 | R5.2 C5.2 22.29,44.96 22.8,44.45
  Top 2.032: C4.+ 22.8,44.45 v22.8,43.88 22.8,35.37 23.56,34.61 U2.56
  Bottom 0.813: v22.8,43.88 25.91,46.99 39.37,46.99 VBAT.1
  pour Top (no thermals): 25.15,35.81 27.05,35.81 27.05,33.4 25.15,33.4
  pour Top (isolate 0.254, no thermals): 23.81,46.99 23.81,45.28 21.78,45.28 21.78,45.91
VBOARD
  Top 1.27: VIN.CH2A VIN.CH1A
  Bottom 1.27: VIN.CH1A 11.81,37.21 24.13,49.53 24.13,52.2 25.02,53.09 33.02,53.09 33.53,52.58 33.53,50.81 J5.3
VDD_EXT  (via drill 0.3 pad 0.41, 0.3 pad 0.61)
  Top 0.254: Q2.4 34.34,13.43 34.64,13.14 35.3,13.14 35.62,13.45 Q2.2 | R8.6 40.12,13.63 40.41,13.34 40.67,13.34 40.96,13.62 R8.5 41.02,13.98 v41.02,15.37 | Q2.2 | v45.59,16.51 44.96,16.51 44.07,17.4 44.07,18.58 U2.15 | Q2.2 35.62,14.79 v36.45,15.62
  Bottom 0.254: J1.9 67.82,11.81 66.93,12.7 63.5,12.7 62.36,13.84 49.4,13.84 47.62,15.62 46.48,15.62 v45.59,16.51 44.45,15.37 v41.02,15.37 40.01,16.38 38.23,16.38 37.47,15.62 v36.45,15.62
VEXT
  Top 1.27: VIN.CH1B VIN.CH2B 2.79,34.16 6.99,29.97 6.99,24.77 9.78,21.97 EXT_PWR.+
VIN  (via drill 0.38 pad 0.81)  (1 unrouted)
  Top 0.305: 50.86,11.49 50.99,11.49 51.69,12.19 60.9,12.19 v60.96,12.26
  Top 0.406: v31.3,36.83 31.3,35.43 33.02,33.72 33.02,24.7 25.15,16.83 25.15,11.87 28.19,8.83 60.39,8.83 v60.96,8.26 60.96,6.73 60.58,6.35 D3.+ D2.+ | R7.2 50.86,11.49 | v50.42,50.86 PWR.+
  Top 0.61: U1.1 U1.2 15.62,41.66 C1.2 C2.2 18.29,36.58 C3.+
  Top 1.27: VIN.COM1 VIN.COM2 | v15.88,36.83 18.67,36.83
  Bottom 0.406: v60.96,8.26 v60.96,12.26 | v15.88,36.83 v31.3,36.83 34.23,36.83 45.34,47.94 49.72,47.94 50.42,48.64 v50.42,50.86
  Bottom 1.27: v15.88,36.83 11.43,32.38 5.97,32.38 5.21,33.15 VIN.COM2
VRTC  (via drill 0.38 pad 0.81)
  Top 0.406: v52.58,32 C6.2 52.32,30.61 U2.26
  Bottom 0.406: J14.+ 37.85,17.27 v52.58,32

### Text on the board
tPlace: PWRKEY | GND | 4.2V | 6 | LNIn_L | (2.8V) | 5 | LNIn_R | 4 | GND | GPIO | 3 | ADC | 2 | PWM2 | 1 | PWM1 | EXT | Xduino | GPRS_TX | GND | RI | Xduino | SWserial | DCD | 2V8 | DSR | TX | GPRS_RX | CTS | NetLight | RX | SWserial | PWRKEY When JP soldered | RTS | DTR | UART(2V8) | Status
bPlace: GPRS/GSM Shield | v1.1 2014/06/06 | www.elecrow.com | 3V CR1220 | SIMHOLDER | SIM Card Holder | 2V8 Logic | DISP_CLK | DISP_DATA | DISP_D/C | 5V Logic | DISP_CS
tNames: J13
